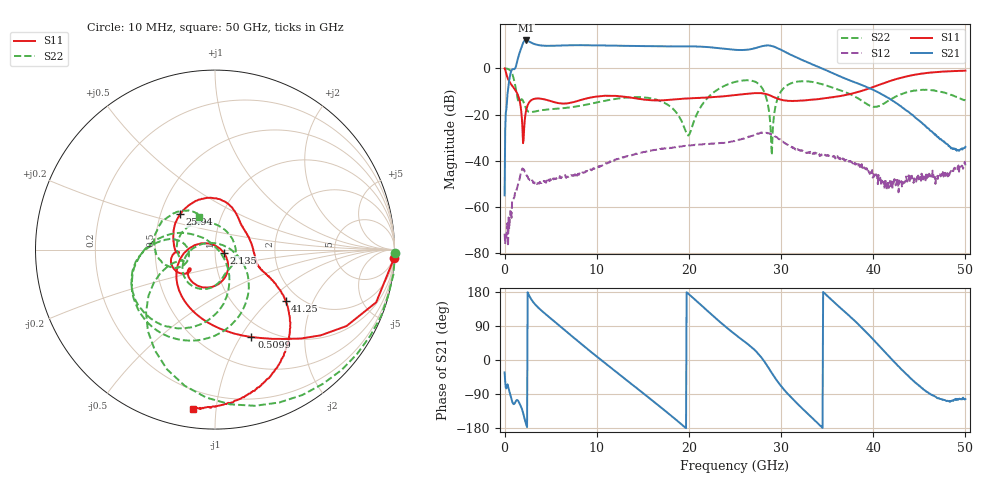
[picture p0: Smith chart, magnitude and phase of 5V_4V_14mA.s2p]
! MARKI MICROWAVE INC.
! Date:  1/07/2020
! Model Number:  APM-6849CH
! Description:  2-port Small Signal S-parameter data for APM-6849CH
! Frequency Range:  10 MHz to 50 GHz
! Port Configuration:  PORT 1: Input
!  PORT 2: Output
! Bias Condition: Vc = +5V, Vb = +4V
! APM-6849CH s2p files are only valid for small signal conditions (below -5 dBm input power)
!S2P File: Measurements: Mag<S11> Ang<S11>, Mag<S21> Ang<S21>, Mag<S12> Ang<S12>, Mag<S22> Ang<S22>!row 1
# Hz S  dB  R 50
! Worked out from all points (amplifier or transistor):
!   801 points, 10 MHz to 50 GHz, reference 50 ohm
!   highest |S21| = 12.2 dB at 2.322 GHz (marker M1)
!   |S21| within 3 dB of that: 1.84 GHz to 22.4 GHz (20.56 GHz wide, 170 % of centre)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
!   unconditionally stable (mu >= 1): 113 MHz to end of sweep
!   at 8.321 GHz: K = 28.52, MAG = 10.4 dB, |S12| = -45.8 dB
!   at 25 GHz: K = 5.08, MAG = 9.7 dB, |S12| = -31.4 dB
!   at 50 GHz: K = 610.75, MAG = -26.9 dB, |S12| = -42.1 dB
!   S11 on the Smith chart (normalised r, x): 10 MHz: 1, -42; 509.9 MHz: 0.83, -1.12; 2.135 GHz: 1.10, -0.04; 25.94 GHz: 0.63, +0.27; 41.25 GHz: 1.69, -1.27; 50 GHz: 0.10, -0.87
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1e7  -0.01 -2.7  -55.13 -32.8  -71.79 -15.2  0.03 -1.2
5.099e8  -5.55 -67.4  -5.03 -80.4  -69.68 -23.3  -0.49 -59.0
1.5097e9  -12.14 -150.2  5.17 -109.0  -49.70 -71.7  -14.34 -161.2
2.134575e9  -25.69 -19.1  11.86 -151.2  -44.18 -148.7  -15.43 115.3
2.322038e9  -18.66 -51.0  12.17 -168.0  -45.72 -162.7  -17.36 82.3
3.071888e9  -13.41 -99.3  10.89 154.1  -49.09 174.6  -18.89 7.4
4.634075e9  -13.75 -137.2  9.84 117.4  -49.46 167.3  -17.80 -38.7
8.383325e9  -13.56 -140.5  10.11 41.2  -45.51 129.8  -16.10 -72.5
1.175765e10  -11.85 -163.5  9.91 -24.6  -40.07 100.9  -13.38 -96.3
1.431964e10  -13.06 -175.8  9.76 -73.8  -37.12 64.3  -12.43 -122.1
1.669416e10  -13.90 -175.5  9.65 -119.7  -35.20 28.7  -13.83 -152.7
2.038092e10  -12.92 177.3  9.57 165.5  -33.35 -29.2  -24.87 20.7
2.269296e10  -12.42 166.0  9.08 115.0  -32.67 -69.5  -10.37 -52.0
2.5005e10  -11.55 147.0  8.11 67.7  -31.42 -112.0  -5.86 -99.1
2.594231e10  -11.15 134.4  8.02 50.4  -30.47 -133.7  -5.18 -119.5
2.825435e10  -10.97 85.2  9.93 -6.2  -27.95 148.9  -11.02 163.5
2.969156e10  -13.21 53.5  8.70 -59.0  -30.46 90.6  -12.40 -72.0
3.131624e10  -14.17 30.6  5.43 -104.2  -34.64 52.5  -6.12 -118.2
3.337832e10  -13.57 3.7  1.79 -153.0  -36.76 18.8  -5.85 -155.2
4.125175e10  -6.25 -36.1  -11.90 21.6  -50.27 141.2  -15.00 -155.2
4.168916e10  -5.63 -38.9  -12.92 10.1  -51.91 112.7  -13.93 -153.8
5e10  -0.96 -97.9  -34.09 -103.1  -42.09 -63.8  -13.81 116.8
